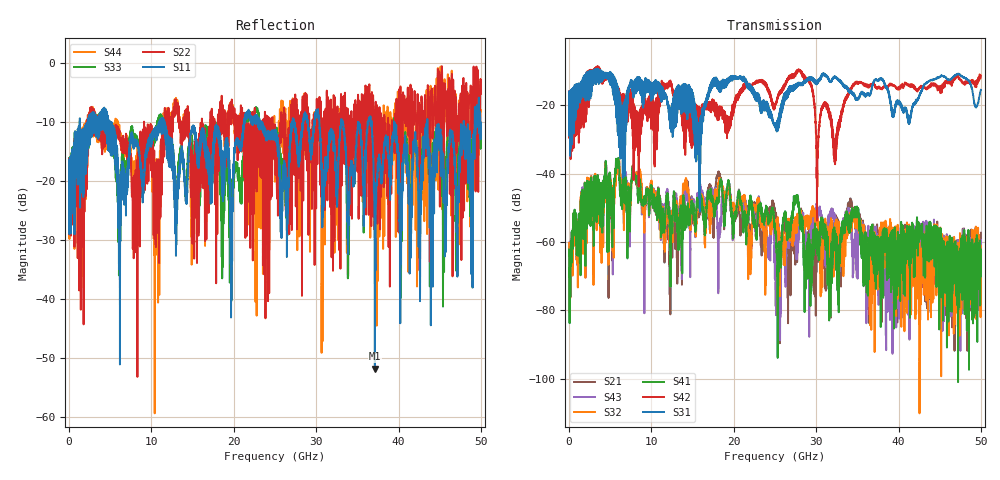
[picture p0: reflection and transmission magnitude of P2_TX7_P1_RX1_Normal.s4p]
!Keysight Technologies,N5225B,MY57041031,A.13.20.10
!Date: Friday, May 31, 2019 11:15:09
!Correction: S11(Full 4 Port(1,2,3,4))
!S12(Full 4 Port(1,2,3,4))
!S13(Full 4 Port(1,2,3,4))
!S14(Full 4 Port(1,2,3,4))
!S21(Full 4 Port(1,2,3,4))
!S22(Full 4 Port(1,2,3,4))
!S23(Full 4 Port(1,2,3,4))
!S24(Full 4 Port(1,2,3,4))
!S31(Full 4 Port(1,2,3,4))
!S32(Full 4 Port(1,2,3,4))
!S33(Full 4 Port(1,2,3,4))
!S34(Full 4 Port(1,2,3,4))
!S41(Full 4 Port(1,2,3,4))
!S42(Full 4 Port(1,2,3,4))
!S43(Full 4 Port(1,2,3,4))
!S44(Full 4 Port(1,2,3,4))
!S4P File: Measurements: <S11,S12,S13,S14>,
!<S21,S22,S23,S24>,
!<S31,S32,S33,S34>,
!<S41,S42,S43,S44>:
# Hz S  dB  R 50.0
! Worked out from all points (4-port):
!   5000 points, 10 MHz to 50 GHz, reference 50 ohm
!   strongest paths, dB at 10 MHz, 12.51 GHz, 25.01 GHz, 37.51 GHz, 50 GHz:
!     S31: -19.6, -21.0, -25.9, -12.8, -15.4
!     S42: -19.4, -14.6, -20.0, -14.9, -11.3
!     S41: -62.2, -54.7, -56.2, -60.5, -68.6
!     S32: -60.3, -52.9, -55.7, -63.6, -61.1
!     S43: -60.1, -51.2, -65.6, -63.3, -60.4
!     S21: -71.9, -56.8, -51.3, -62.4, -57.3
!   lowest |S11| = -51.9 dB at 37.13 GHz (marker M1), VSWR 1.01, Z = 50.2 + j0.0566 ohm
!   |S11| at or under -10 dB: 4.96 GHz to 11.03 GHz (6.066 GHz wide, 75.9 % of centre); 11.57 GHz to 21.26 GHz (9.683 GHz wide, 59 % of centre); 36.74 GHz to 43.5 GHz (6.759 GHz wide, 16.8 % of centre)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
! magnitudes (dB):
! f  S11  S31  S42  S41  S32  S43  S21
! 10 MHz  -20.2  -19.6  -19.4  -62.2  -60.3  -60.1  -71.9
! 5.9 GHz  -17.2  -17.7  -15.4  -37.0  -37.8  -37.4  -37.4
! 12.32 GHz  -12.8  -21.7  -13.6  -73.1  -58.9  -57.5  -57.9
! 18.17 GHz  -11.6  -15.3  -21.4  -47.6  -43.4  -58.8  -39.4
! 25.59 GHz  -21.5  -22.5  -16.6  -64.8  -75.9  -62.0  -89.6
! 37.13 GHz  -51.9  -12.4  -14.2  -60.1  -63.6  -60.3  -60.6
! 50 GHz  -11.1  -15.4  -11.3  -68.6  -61.1  -60.4  -57.3
